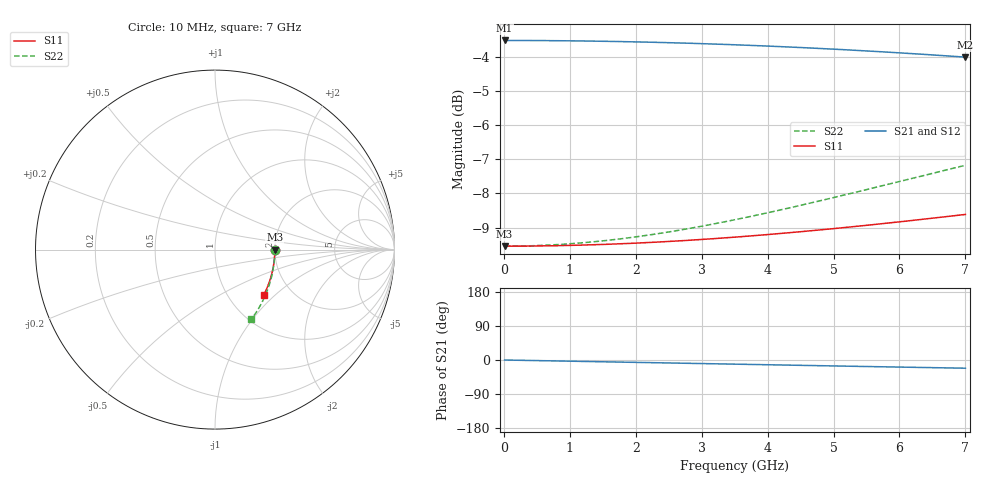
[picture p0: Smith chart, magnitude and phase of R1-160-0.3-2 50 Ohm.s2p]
!version-2
!date-03.2021
# MHz S RI R 50
!Freq ReS11 ImS11 ReS21 ImS21 ReS12 ImS12 ReS22 ImS22
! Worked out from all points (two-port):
!   700 points, 10 MHz to 7 GHz, reference 50 ohm
!   highest |S21| = -3.52 dB at 10 MHz (marker M1); lowest = -4.0 dB at 7 GHz (marker M2)
!   |S21| within 3 dB of the highest: start of sweep to end of sweep
!   lowest |S11| = -9.5 dB at 10 MHz (marker M3), VSWR 2.00, Z = 100 - j0.0868 ohm
!   |S11| at or under -10 dB: nowhere
!   |S22| runs from -9.5 to -7.2 dB; largest |S21 - S12| = 0
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10  0.3333 -0.000386  0.6667 -0.00037  0.6667 -0.00037  0.3333 -0.000615
40  0.3333 -0.00154  0.6667 -0.00148  0.6667 -0.00148  0.3333 -0.00246
310  0.3332 -0.012  0.6665 -0.0115  0.6665 -0.0115  0.333 -0.0191
590  0.3329 -0.0227  0.666 -0.0218  0.666 -0.0218  0.3323 -0.0362
880  0.3323 -0.0339  0.6653 -0.0325  0.6653 -0.0325  0.331 -0.054
1180  0.3314 -0.0454  0.6641 -0.0436  0.6641 -0.0436  0.3292 -0.0723
1460  0.3304 -0.0561  0.6628 -0.0538  0.6628 -0.0538  0.3271 -0.0893
1750  0.3292 -0.0672  0.6611 -0.0644  0.6611 -0.0644  0.3243 -0.1069
2040  0.3277 -0.0782  0.6591 -0.0748  0.6591 -0.0748  0.3211 -0.1243
2340  0.3259 -0.0895  0.6568 -0.0856  0.6568 -0.0856  0.3173 -0.1422
2630  0.324 -0.1004  0.6542 -0.0959  0.6542 -0.0959  0.3132 -0.1593
2920  0.3219 -0.1112  0.6514 -0.106  0.6514 -0.106  0.3086 -0.1762
3210  0.3195 -0.122  0.6483 -0.1161  0.6483 -0.1161  0.3035 -0.193
3510  0.3169 -0.133  0.6447 -0.1264  0.6447 -0.1264  0.2978 -0.2101
4080  0.3113 -0.1536  0.6373 -0.1455  0.6373 -0.1455  0.2858 -0.242
4670  0.3047 -0.1746  0.6286 -0.1646  0.6286 -0.1646  0.2717 -0.274
5250  0.2975 -0.1947  0.6192 -0.1827  0.6192 -0.1827  0.2563 -0.3044
5840  0.2895 -0.2147  0.6087 -0.2003  0.6087 -0.2003  0.2392 -0.334
6180  0.2846 -0.2259  0.6022 -0.2101  0.6022 -0.2101  0.2288 -0.3505
6510  0.2797 -0.2367  0.5958 -0.2194  0.5958 -0.2194  0.2182 -0.3661
6950  0.2728 -0.2507  0.5868 -0.2313  0.5868 -0.2313  0.2036 -0.3862
7000  0.272 -0.2523  0.5858 -0.2326  0.5858 -0.2326  0.2019 -0.3885
